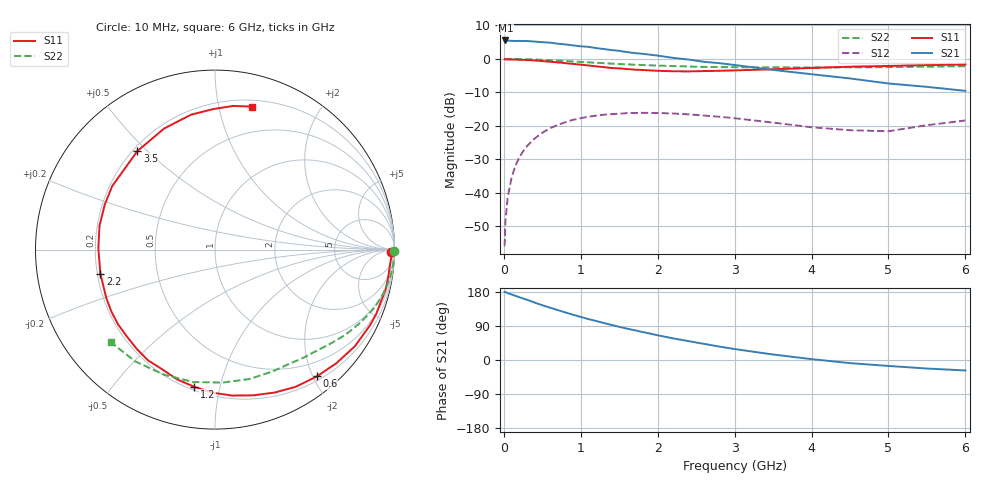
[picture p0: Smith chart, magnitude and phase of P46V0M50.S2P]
! SIEMENS Small Signal Semiconductors
! BFP182
! Si NPN RF Bipolar Junction Transistor in SOT143
! VCE = 6 V  IC = 0.5 mA
! Common Emitter S-Parameters:  March  1996
# GHz  S  MA  R  50
!  f  S11  S21  S12  S22
! GHz  MAG  ANG  MAG  ANG  MAG  ANG  MAG  ANG
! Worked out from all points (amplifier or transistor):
!   36 points, 10 MHz to 6 GHz, reference 50 ohm
!   highest |S21| = 5.5 dB at 20 MHz (marker M1)
!   |S21| within 3 dB of that: start of sweep to 1.456 GHz
!   unconditionally stable (mu >= 1): 2.996 GHz to end of sweep
!   at 250 MHz: K = 0.09, MSG = 16.5 dB, |S12| = -27.6 dB
!   at 1.4 GHz: K = 0.49, MSG = 9.6 dB, |S12| = -16.5 dB
!   at 6 GHz: K = 1.21, MAG = 1.6 dB, |S12| = -18.4 dB
!   S11 on the Smith chart (normalised r, x): 10 MHz: 76, -53; 600 MHz: 0.26, -2.06; 1.2 GHz: 0.22, -0.83; 2.2 GHz: 0.21, -0.10; 3.5 GHz: 0.22, +0.47; 6 GHz: 0.26, +1.26
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0.01  0.9824 -0.7  1.867 179.7  0.0016 88.8  0.999 -0.3
0.02  0.985 -1.8  1.882 179.3  0.0037 86.7  0.997 -0.6
0.05  0.9793 -4.5  1.87 176.4  0.0086 89.1  0.9981 -1.5
0.1  0.9771 -8.6  1.857 173.0  0.0167 83.2  0.9961 -3.1
0.15  0.9763 -13.1  1.845 169.4  0.0254 81.2  0.9958 -4.6
0.2  0.969 -17.5  1.853 165.6  0.0336 79.0  0.9936 -6.2
0.3  0.9612 -26.0  1.848 159.1  0.0497 72.9  0.9867 -9.3
0.4  0.9473 -34.6  1.81 151.5  0.0648 67.6  0.9779 -12.2
0.6  0.9062 -51.2  1.747 138.1  0.092 56.8  0.9545 -17.9
0.8  0.8629 -67.4  1.644 125.5  0.1134 46.9  0.9275 -23.0
1.1  0.7967 -91.3  1.511 108.0  0.137 33.7  0.8866 -29.8
1.2  0.7728 -98.7  1.448 102.9  0.142 29.4  0.8738 -32.0
1.6  0.7047 -128.1  1.262 82.8  0.1548 15.8  0.8286 -39.4
2  0.6633 -155.8  1.118 65.2  0.1554 4.8  0.7925 -46.3
2.2  0.6527 -168.2  1.035 57.1  0.1529 -0.2  0.7813 -49.9
2.8  0.6632 157.7  0.863 35.4  0.1369 -11.1  0.7538 -60.6
3.5  0.699 128.2  0.684 14.5  0.1118 -17.0  0.7461 -75.1
4  0.7318 112.7  0.59 2.3  0.0953 -13.7  0.7423 -86.8
4.5  0.7632 100.1  0.51 -8.3  0.086 -6.7  0.7476 -99.4
5  0.7832 90.7  0.429 -15.7  0.0831 8.0  0.7526 -112.3
5.5  0.8069 82.7  0.382 -22.5  0.1023 14.7  0.7653 -125.6
6  0.8233 75.4  0.333 -27.7  0.1203 16.0  0.7771 -138.5
